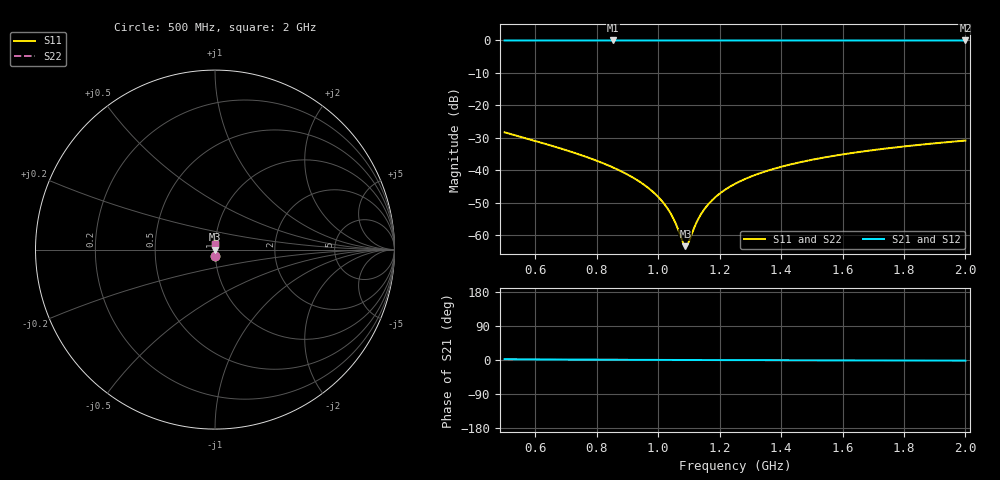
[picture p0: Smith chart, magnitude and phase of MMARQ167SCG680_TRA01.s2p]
! MMARQ167SCG680_TRA01  S-PARAMETER MODEL  ( General Type )
! Model Generated by TAIYO YUDEN Corporation (http://www.ty-top.com)
! Version 1.0
! TAIYO YUDEN Control No. 150305
! Copyright(c) 2015 TAIYO YUDEN CO.,LTD. All Rights Reserved.
! Product Description (link to TY-COMPAS)
! https://ds.yuden.co.jp/TYCOMPAS/or/detail?pn=MMARQ167SCG680JTRA01&u=M
! Products Name : Multilayer Ceramic Capacitors
! Characteristics :
!  Capacitance : 68 pF , Rated Voltage : 250V , TCC : CG / C0G
!  Case Size : 1.6 x 0.8 / 0.063 x 0.031 [mm/inch] , Thickness : 0.7 / 0.028 [mm/inch]
!  (Conditions: Temperature = 25 degC , DC Bias Current/Voltage = 0A / 0V)
! External Node Assignments :
!  1  o---| |---o  2
! GND o---------o GND
! Frequency Range : 500MHz  -  2GHz  [ 401 STEP ]
# MHz S RI R 50
! Freq[MHz].  S11 Real  S11 Imag  S21 Real  S21 Imag  S12 Real  S12 Imag  S22 Real  S22 Imag
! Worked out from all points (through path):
!   401 points, 500 MHz to 2 GHz, reference 50 ohm
!   highest |S21| = -0.01 dB at 852.5 MHz (marker M1); lowest = 0.0 dB at 2 GHz (marker M2)
!   lowest |S11| = -63.4 dB at 1.089 GHz (marker M3), VSWR 1.00, Z = 50.1 - j0.00431 ohm
!   |S11| at or under -10 dB: start of sweep to end of sweep
!   |S22| runs from -63.4 to -28.3 dB; largest |S21 - S12| = 0
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500  0.00181 -0.0384  0.9982 0.0384  0.9982 0.0384  0.00181 -0.0384
751.25  0.000751 -0.017  0.9992 0.017  0.9992 0.017  0.000751 -0.017
852.5  0.000644 -0.0111  0.9994 0.0111  0.9994 0.0111  0.000644 -0.0111
938.75  0.00062 -0.00668  0.9994 0.00668  0.9994 0.00668  0.00062 -0.00668
972.5  0.000623 -0.00509  0.9994 0.00509  0.9994 0.00509  0.000623 -0.00509
1002.5  0.000631 -0.00373  0.9994 0.00373  0.9994 0.00373  0.000631 -0.00373
1021.25  0.000638 -0.0029  0.9994 0.0029  0.9994 0.0029  0.000638 -0.0029
1040  0.000647 -0.00208  0.9994 0.00208  0.9994 0.00208  0.000647 -0.00208
1055  0.000655 -0.00145  0.9993 0.00145  0.9993 0.00145  0.000655 -0.00145
1081.25  0.000671 -0.000351  0.9993 0.000351  0.9993 0.000351  0.000671 -0.000351
1088.75  0.000676 -4.3e-05  0.9993 4.3e-05  0.9993 4.3e-05  0.000676 -4.3e-05
1096.25  0.000681 0.000263  0.9993 -0.000263  0.9993 -0.000263  0.000681 0.000263
1130  0.000708 0.00161  0.9993 -0.00161  0.9993 -0.00161  0.000708 0.00161
1156.25  0.000732 0.00264  0.9993 -0.00264  0.9993 -0.00264  0.000732 0.00264
1197.5  0.000773 0.0042  0.9992 -0.0042  0.9992 -0.0042  0.000773 0.0042
1250  0.000834 0.00612  0.9992 -0.00612  0.9992 -0.00612  0.000834 0.00612
1298.75  0.000896 0.00785  0.9991 -0.00785  0.9991 -0.00785  0.000896 0.00785
1355  0.000977 0.00977  0.999 -0.00977  0.999 -0.00977  0.000977 0.00977
1501.25  0.00122 0.0145  0.9988 -0.0145  0.9988 -0.0145  0.00122 0.0145
1617.5  0.00144 0.018  0.9986 -0.018  0.9986 -0.018  0.00144 0.018
1752.5  0.00173 0.0219  0.9983 -0.0219  0.9983 -0.0219  0.00173 0.0219
2000  0.00235 0.0286  0.9977 -0.0286  0.9977 -0.0286  0.00235 0.0286
